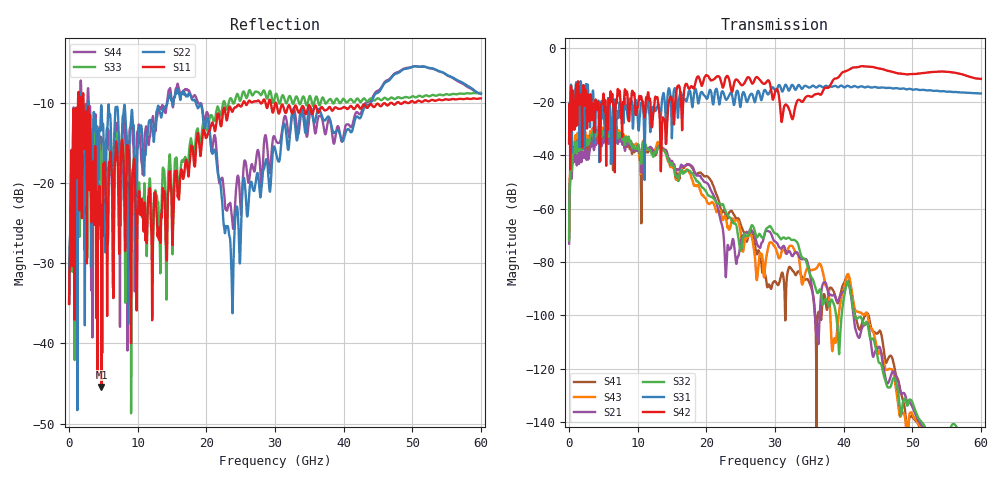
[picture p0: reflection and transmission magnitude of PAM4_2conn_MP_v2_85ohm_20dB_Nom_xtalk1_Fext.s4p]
! Info: Touchstone file created by Circ.  Input file=FAB50GbE_2conn_Midplane_Examax_Topo2_v2_85ohm_20dB_Nom.circ
# Hz S RI R 50
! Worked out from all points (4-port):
!   6000 points, 10 MHz to 60 GHz, reference 50 ohm
!   strongest paths, dB at 10 MHz, 15.01 GHz, 30.01 GHz, 45.01 GHz, 60 GHz:
!     S42: -35.6, -19.6, -16.3, -7.5, -11.4
!     S31: -35.5, -31.3, -15.8, -14.7, -16.9
!     S32: -71.9, -43.2, -69.2, -116.5, -151.2
!     S21: -73.1, -42.2, -72.3, -112.0, -146.7
!     S43: -71.2, -44.4, -74.4, -114.0, -155.3
!     S41: -68.6, -43.2, -87.2, -106.6, -155.9
!   lowest |S11| = -45.4 dB at 4.72 GHz (marker M1), VSWR 1.01, Z = 50.5 + j0.00631 ohm
!   |S11| at or under -10 dB: start of sweep to 1.299 GHz; 2.113 GHz to 25.32 GHz (23.2 GHz wide, 169 % of centre); 30.17 GHz to 45.88 GHz (15.71 GHz wide, 41.3 % of centre)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
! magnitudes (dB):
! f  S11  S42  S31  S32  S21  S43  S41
! 10 MHz  -35.0  -35.6  -35.5  -71.9  -73.1  -71.2  -68.6
! 760 MHz  -15.4  -30.3  -20.9  -38.7  -42.4  -37.0  -39.5
! 4.72 GHz  -45.4  -20.7  -20.1  -33.1  -36.7  -31.3  -34.1
! 20.23 GHz  -13.8  -10.3  -18.1  -55.0  -50.7  -58.0  -48.0
! 27.39 GHz  -9.8  -10.8  -16.6  -70.8  -73.3  -86.5  -77.0
! 32.51 GHz  -11.3  -26.5  -13.7  -71.7  -77.8  -74.0  -83.0
! 60 GHz  -9.4  -11.4  -16.9  -151.2  -146.7  -155.3  -155.9
